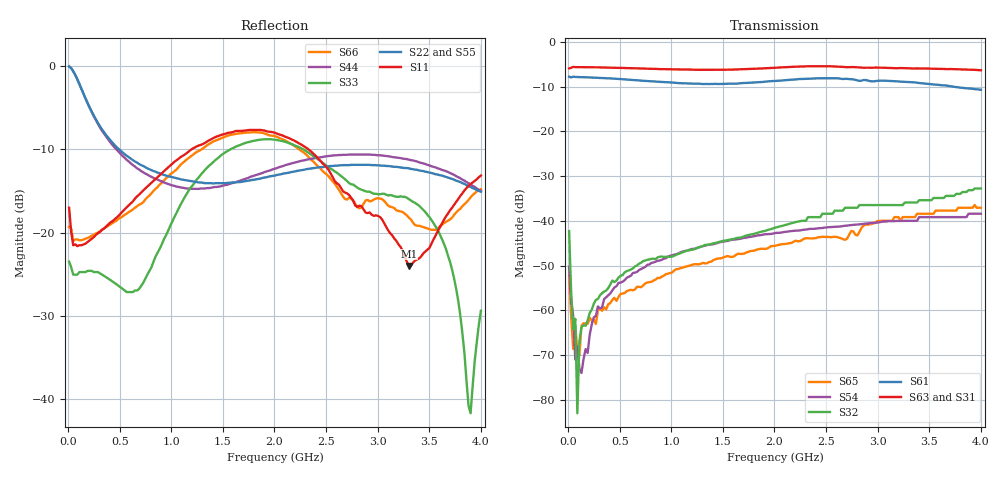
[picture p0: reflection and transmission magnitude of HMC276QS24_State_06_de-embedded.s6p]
! Hittite Microwave Corporation
! 20 Alpha Road
! Chelmsford, MA 01824
! Tel: 978-250-3343
! Fax: 978-250-3373
! Device: HMC276QS24, 0.7-3.0 GHz, GaAS MMIC 4x2 Switch Matrix in 24-lead QSOP package
! Misc: Data was de-embedded to package pins.
!  Port 1 = OP1
!  Port 2 = VL
!  Port 3 = VH
!  Port 4 = HH
!  Port 5 = HL
!  Port 6 = OP2
!  Vdd = +5 V
!  Vctl = 0 V[Logic 0] / +5 V[Logic 1]
!  State 06,  VH to OP1,  VH to OP2
!  Control Lines (Logic)
!  HV 1 = 0, Tone 1 = 1
!  HV 2 = 0, Tone 2 = 1
!  Data reformated to new Touchstone file format - Wed Jan 10 15:12:41 2007
# MHz S DB R 50
! 6 Port Network Data
! freq  dbS11  angS11  dbS12  angS12  dbS13  angS13  dbS14  angS14
!  dbS15  angS15  dbS16  angS16
!  dbS21  angS21  dbS22  angS22
!  dbS23  angS23  dbS24  angS24  dbS25  angS25  dbS26  angS26
!  dbS31  angS31  dbS32  angS32  dbS33  angS33  dbS34  angS34
!  dbS35  angS35  dbS36  angS36
!  dbS41  angS41  dbS42  angS42
!  dbS43  angS43  dbS44  angS44  dbS45  angS45  dbS46  angS46
!  dbS51  angS51  dbS52  angS52  dbS53  angS53  dbS54  angS54
!  dbS55  angS55  dbS56  angS56
!  dbS61  angS61  dbS62  angS62
!  dbS63  angS63  dbS64  angS64  dbS65  angS65  dbS66  angS66
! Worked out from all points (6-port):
!   201 points, 10 MHz to 4 GHz, reference 50 ohm
!   strongest paths, dB at 10 MHz, 1.008 GHz, 2.005 GHz, 3.002 GHz, 4 GHz:
!     S63: -5.9, -6.1, -5.8, -5.7, -6.3
!     S31: -6.0, -6.4, -6.0, -5.8, -6.4
!     S61: -7.8, -9.1, -8.8, -8.7, -10.7
!     S32: -42.3, -48.0, -41.5, -36.5, -32.8
!     S54: -50.3, -47.7, -42.7, -40.4, -38.4
!     S65: -52.3, -51.6, -45.6, -40.0, -37.1
!   lowest |S11| = -24.0 dB at 3.302 GHz (marker M1), VSWR 1.13, Z = 54 + j5.17 ohm
!   |S11| at or under -10 dB: start of sweep to 1.198 GHz; 2.329 GHz to end of sweep
